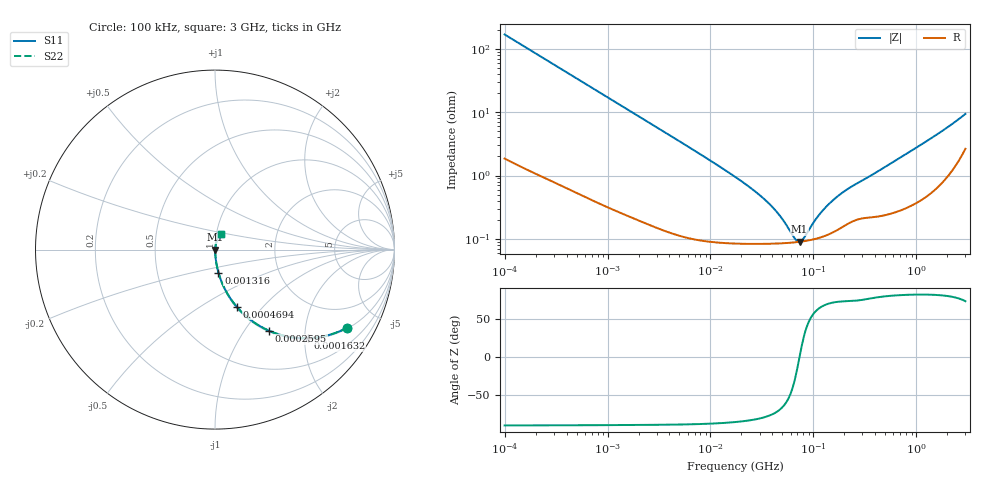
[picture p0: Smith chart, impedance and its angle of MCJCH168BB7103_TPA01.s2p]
! MCJCH168BB7103_TPA01  S-PARAMETER MODEL  ( Standard Model )
! Model Generated by TAIYO YUDEN Corporation (http://www.ty-top.com)
! Version 1.0
! TAIYO YUDEN Control No. 220601
! Copyright(c) 2015 TAIYO YUDEN CO.,LTD. All Rights Reserved.
! Product Description (link to TY-COMPAS)
! https://ds.yuden.co.jp/TYCOMPAS/or/detail?pn=MCJCH168BB7103KTPA01&u=M
! Products Name : Multilayer Ceramic Capacitors
! Characteristics :
!  Capacitance : 0.01 [uF] , Rated Voltage : 100 [V] , TCC : X7R
!  Case Size : 1.6 x 0.8 / 0.063 x 0.031 [mm/inch] , Thickness : 0.8 / 0.031 [mm/inch]
!  (Conditions: Temperature = 25 [degC] , DC Bias Voltage = 0 [V])
! External Node Assignments :
!  1  o---| |---o  2
! GND o---------o GND
! Frequency Range : 100kHz  -  3GHz  [ 401 STEP ]
# MHZ S RI R 50
! Freq[MHz].  S11 Real  S11 Imag  S21 Real  S21 Imag  S12 Real  S12 Imag  S22 Real  S22 Imag
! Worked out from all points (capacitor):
!   401 points, 100 kHz to 3 GHz, reference 50 ohm
!   read as one part in series: C = 9.42 nF near 105.3 kHz
!   lowest |Z| = 90 mohm at 73.34 MHz (marker M1)
!   series resonance near 73.24 MHz, so ESL is about 500 pH
!   S11 on the Smith chart (normalised r, x): 100 kHz: 1.04, -3.37; 163.2 kHz: 1.02, -2.07; 259.5 kHz: 1.02, -1.31; 469.4 kHz: 1.01, -0.73; 1.316 MHz: 1.01, -0.26; 3 GHz: 1.05, +0.18
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0.1  0.7375 -0.4345  0.2625 0.4345  0.2625 0.4345  0.7375 -0.4345
0.163179  0.5179 -0.4937  0.4821 0.4937  0.4821 0.4937  0.5179 -0.4937
0.259498  0.3022 -0.4526  0.6978 0.4526  0.6978 0.4526  0.3022 -0.4526
0.344552  0.1996 -0.3926  0.8004 0.3926  0.8004 0.3926  0.1996 -0.3926
0.469427  0.1205 -0.3179  0.8795 0.3179  0.8795 0.3179  0.1205 -0.3179
0.562235  0.0883 -0.2758  0.9117 0.2758  0.9117 0.2758  0.0883 -0.2758
1.316074  0.0193 -0.128  0.9807 0.128  0.9807 0.128  0.0193 -0.128
3.161081  0.00444 -0.0546  0.9956 0.0546  0.9956 0.0546  0.00444 -0.0546
17.7727  0.000928 -0.00925  0.9991 0.00925  0.9991 0.00925  0.000928 -0.00925
27.54426  0.000862 -0.00545  0.9991 0.00545  0.9991 0.00545  0.000862 -0.00545
37.52708  0.000849 -0.00344  0.9992 0.00344  0.9992 0.00344  0.000849 -0.00344
48.55934  0.000854 -0.00202  0.9991 0.00202  0.9991 0.00202  0.000854 -0.00202
66.15861  0.000882 -0.000486  0.9991 0.000486  0.9991 0.000486  0.000882 -0.000486
73.34282  0.000899 6.66e-06  0.9991 -6.66e-06  0.9991 -6.66e-06  0.000899 6.66e-06
81.30716  0.00092 0.000499  0.9991 -0.000499  0.9991 -0.000499  0.00092 0.000499
97.38194  0.000974 0.00138  0.999 -0.00138  0.999 -0.00138  0.000974 0.00138
126.0104  0.0011 0.0027  0.9989 -0.0027  0.9989 -0.0027  0.0011 0.0027
176.1623  0.00144 0.00463  0.9986 -0.00463  0.9986 -0.00463  0.00144 0.00463
227.9507  0.00184 0.00623  0.9982 -0.00623  0.9982 -0.00623  0.00184 0.00623
547.5153  0.00267 0.0148  0.9973 -0.0148  0.9973 -0.0148  0.00267 0.0148
1457.883  0.00718 0.0398  0.9928 -0.0398  0.9928 -0.0398  0.00718 0.0398
3000  0.0332 0.0849  0.9668 -0.0849  0.9668 -0.0849  0.0332 0.0849
